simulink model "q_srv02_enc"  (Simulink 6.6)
settings: Solver=FixedStepDiscrete  StartTime=0.0  StopTime=inf  FixedStep=0.002  RelTol=1e-3  AbsTol=1e-6
undefined symbols (not defined in the file or in its folder): HIL, qc_get_step_size
libraries: quarc_library x4, simulink x1

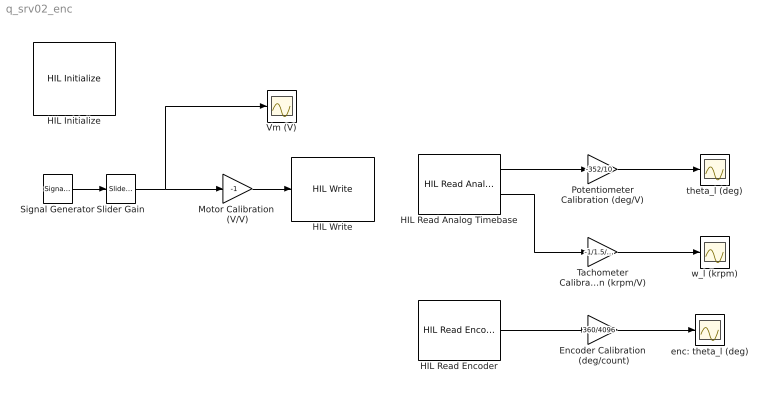
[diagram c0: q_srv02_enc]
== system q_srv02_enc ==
  Encoder Calibration  (deg/count) : Gain  Gain=360/4096
  HIL Initialize : quarc_library/Data Acquisition/Generic/Configuration/HIL Initialize  object_name=HIL-1  board_type=q8  board_number=0  exclusive=off  active=off  hardware_clocks=[0:1]  clock_modes=[0 0]  set_clock_params_at_start=on  set_clock_params_at_switch_in=off  analog_input_channels=[0:7]  analog_input_maximums=10  analog_input_minimums=-10  set_analog_input_params_at_start=off  set_analog_input_params_at_switch_in=off  analog_output_channels=[0:7]  analog_output_maximums=[10]  analog_output_minimums=[-10]  initial_analog_outputs=[0]  final_analog_outputs=[0]  watchdog_analog_outputs=0  set_analog_output_params_at_start=on  set_analog_output_params_at_switch_in=off  set_analog_outputs_at_start=on  set_analog_outputs_at_switch_in=off  set_analog_outputs_at_terminate=on  set_analog_outputs_at_switch_out=off  set_analog_outputs_on_watchdog=off  digital_input_channels=[]  digital_output_channels=[]  digital_output_configuration=[]  initial_digital_outputs=[1]  final_digital_outputs=[1]  watchdog_digital_outputs=[2]  set_digital_output_params_at_start=off  set_digital_output_params_at_switch_in=off  set_digital_outputs_at_start=on  set_digital_outputs_at_switch_in=off  set_digital_outputs_at_terminate=on  set_digital_outputs_at_switch_out=off  set_digital_outputs_on_watchdog=off  encoder_channels=[0:7]  quadrature=[4]  encoder_filter_frequency=(1/120e-9)/1  initial_encoder_counts=[0]  set_encoder_params_at_start=on  set_encoder_params_at_switch_in=off  set_encoder_counts_at_start=on  set_encoder_counts_at_switch_in=off  pwm_channels=[]  pwm_modes=[0]  pwm_frequency=(1/60e-9)/1024  pwm_configuration=[]  pwm_alignment=[]  pwm_polarity=[]  pwm_leading_deadband=[]  pwm_trailing_deadband=[]  initial_pwm_outputs=[0]  final_pwm_outputs=[0]  watchdog_pwm_outputs=[]  set_pwm_params_at_start=on  set_pwm_params_at_switch_in=off  set_pwm_outputs_at_start=on  set_pwm_outputs_at_switch_in=off  set_pwm_outputs_at_terminate=on  set_pwm_outputs_at_switch_out=off  set_pwm_outputs_on_watchdog=off  other_output_channels=[]  initial_other_outputs=[]  final_other_outputs=[]  watchdog_other_outputs=[]  set_other_outputs_at_start=off  set_other_outputs_at_switch_in=off  set_other_outputs_at_terminate=off  set_other_outputs_at_switch_out=off  set_other_outputs_on_watchdog=off
  HIL Read Analog Timebase : quarc_library/Data Acquisition/Generic/Timebases/HIL Read Analog Timebase  object_name=HIL-1  clock=0  channels=[0:1]  samples_in_buffer=max(ceil(1/qc_get_step_size), 1)  active=on  vector_output=off
  HIL Read Encoder : quarc_library/Data Acquisition/Generic/Immediate I//O/HIL Read Encoder  object_name=HIL-1  channels=0  sample_time=qc_get_step_size  active=on  vector_output=off  data_type_mode=Inherit via back propagation  data_type=double
  HIL Write : quarc_library/Data Acquisition/Generic/Immediate I//O/HIL Write  Tag=unassigned  object_name=HIL-1  analog_channels=0  pwm_channels=[]  digital_channels=[]  other_channels=[]  sample_time=-1  active=off  vector_input=off
  Motor Calibration  (V/V) : Gain  Gain=-1
  Potentiometer Calibration (deg/V) : Gain  Gain=-352/10
  Signal Generator : SignalGenerator
  Slider Gain : simulink/Math Operations/Slider Gain  SystemSampleTime=-1  low=0  gain=1  high=2
  Tachometer Calibration (krpm/V) : Gain  Gain=-1/1.5/70
  Vm (V) : Scope
  enc: theta_l (deg) : Scope
  theta_l (deg) : Scope
  w_l (krpm) : Scope
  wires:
  Signal Generator/1 -> Slider Gain/1
  Slider Gain/1 -> Vm (V)/1, Motor Calibration  (V/V)/1
  HIL Read Analog Timebase/1 -> Potentiometer Calibration (deg/V)/1
  Motor Calibration  (V/V)/1 -> HIL Write/1
  Potentiometer Calibration (deg/V)/1 -> theta_l (deg)/1
  Tachometer Calibration (krpm/V)/1 -> w_l (krpm)/1
  Encoder Calibration  (deg/count)/1 -> enc: theta_l (deg)/1
  HIL Read Analog Timebase/2 -> Tachometer Calibration (krpm/V)/1
  HIL Read Encoder/1 -> Encoder Calibration  (deg/count)/1
